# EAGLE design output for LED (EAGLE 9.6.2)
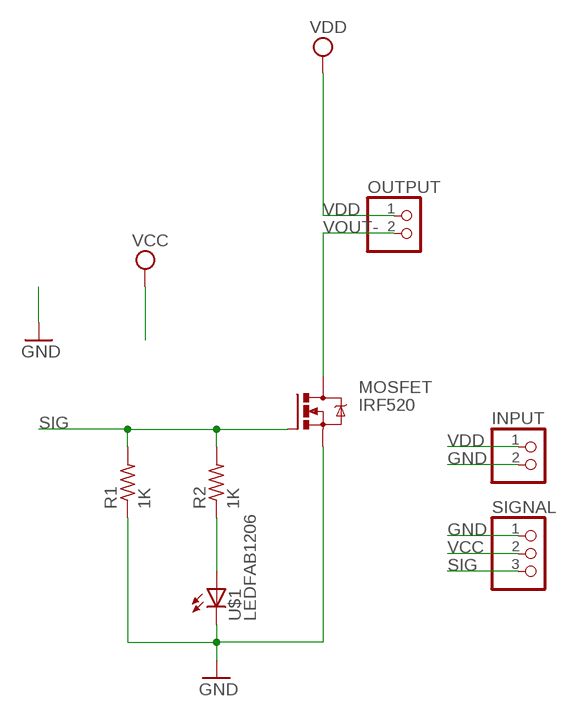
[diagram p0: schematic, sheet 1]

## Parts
INPUT  PINHD-1X2  [1X02]
MOSFET  IRF520  [TO220BV]
OUTPUT  PINHD-1X2  [1X02]
R1  1K  R1206FAB  [R1206FAB]
R2  1K  R1206FAB  [R1206FAB]
SIGNAL  PINHD-1X3  [1X03]
U$1  LEDFAB1206  [LED1206FAB]

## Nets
GND: INPUT.2 SIGNAL.1
N$4: R2.1 U$1.1(A)
SIG: MOSFET.G R1.2 R2.2 SIGNAL.3
VCC: SIGNAL.2
VDD: INPUT.1 OUTPUT.1
VOUT-: MOSFET.D MOSFET.S OUTPUT.2 R1.1 U$1.2(C) ; supply symbol labelled GND

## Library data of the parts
INPUT OUTPUT = pinhead:PINHD-1X2: PIN HEADER
MOSFET = transistor-power:IRF520: HEXFET Power MOSFET
R1 R2 = fab:R: Resistor (US Symbol)
SIGNAL = pinhead:PINHD-1X3: PIN HEADER
U$1 = fab:LED: LED

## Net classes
0 default: width 0.406 mm, clearance 0.406 mm

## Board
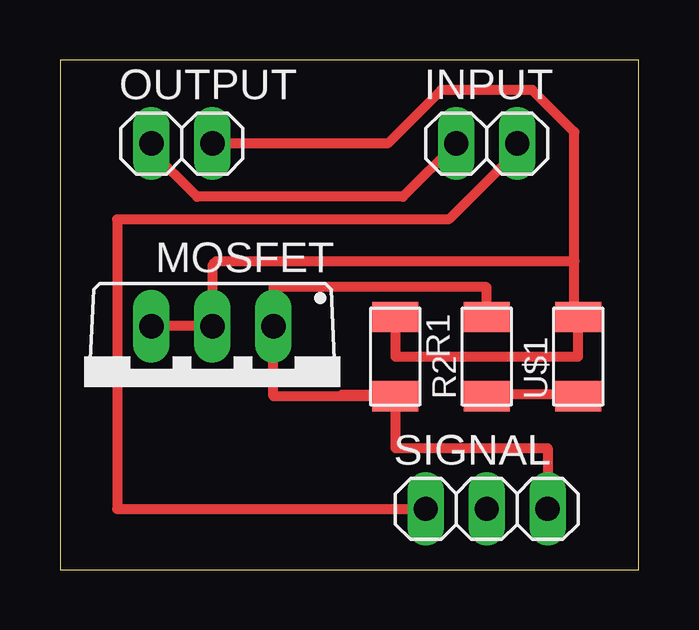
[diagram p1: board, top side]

Size 24.11 x 21.26 mm. Coordinates in mm from the lower left corner, seen from the top.
Outline: 0,0 24.11,0 24.11,21.26 0,21.26 0,0
Copper layers (1*16): Top 0.035mm / dielectric 1.5mm / Bottom 0.035mm
Design rules "default": minimum track width 6mil, minimum drill 0.35mm, track to track 6mil, track to pad 6mil, pad to pad 6mil, via to via 6mil, smd to smd 6mil, copper to edge 40mil, drill to drill 6mil, minimum pad ring 10mil, minimum via ring 8mil, stop-mask expansion 4mil, vias tented up to drill 0mil, thermal gap 10mil

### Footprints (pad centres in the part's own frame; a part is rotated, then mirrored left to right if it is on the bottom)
1X02 = drill 1.016 long: 1 -1.27,0; 2 1.27,0
TO220BV = drill 1.016 long: D 0,-2.54; G -2.54,-2.54; S 2.54,-2.54
R1206FAB = smd 1.27 x 1.905: 1 -1.651,0; 2 1.651,0
1X03 = drill 1.016 long: 1 -2.54,0; 2 0,0; 3 2.54,0
LED1206FAB = smd 1.27 x 1.905: 1 -1.651,0; 2 1.651,0

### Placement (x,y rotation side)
INPUT  17.78,17.78 0 top
MOSFET  6.35,7.62 180 top
OUTPUT  5.08,17.78 0 top
R1  13.97,8.89 270 top
R2  17.78,8.89 90 top
SIGNAL  17.78,2.54 0 top
U$1  21.59,8.89 90 top

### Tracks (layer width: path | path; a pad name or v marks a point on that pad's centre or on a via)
GND
  Top 0.406: 8.57,2.54 SIGNAL.1 2.38,2.54 2.38,14.61 16.19,14.61 19.05,17.46 INPUT.2
N$4
  Top 0.406: R2.1 17.78,7.3 21.59,7.3 U$1.1
SIG
  Top 0.406: 11.75,7.3 13.97,7.3 R1.2 | R1.2 8.89,7.24 MOSFET.G 8.89,11.79 17.78,11.79 R2.2 | R1.2 13.97,5.08 20.32,5.08 SIGNAL.3
VDD
  Top 0.406: OUTPUT.1 3.81,17.46 5.71,15.56 14.29,15.56 INPUT.1
VOUT-
  Top 0.406: MOSFET.S MOSFET.D 6.35,12.7 6.51,12.86 21.43,12.86 | OUTPUT.2 13.65,17.78 15.88,20 19.68,20 21.43,18.26 21.43,12.86 | 21.43,12.86 21.43,10.64 U$1.2 21.59,8.89 13.97,8.89 R1.1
